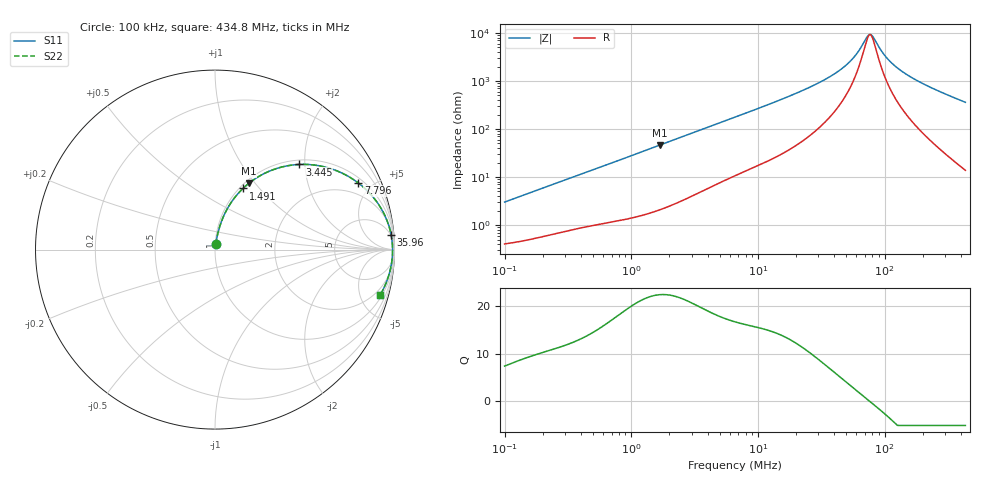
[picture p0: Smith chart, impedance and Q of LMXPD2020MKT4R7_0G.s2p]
! LMXPD2020MKT4R7_0G  S-PARAMETER MODEL  ( General Type )
! Model Generated by TAIYO YUDEN Corporation (http://www.ty-top.com)
! Version 1.0
! TAIYO YUDEN Control No. 191023NI43SB-FBB
! Copyright(c) 2019 TAIYO YUDEN CO.,LTD. All Rights Reserved.
! Product Description (link to TY-COMPAS)
! https://ds.yuden.co.jp/TYCOMPAS/or/detail?pn=LMXPD2020MKT4R7M0G&u=M
! Products Name : Inductors
! Characteristics :
!  Inductance : 4.7 uH , SRF(min) : -Hz , DC Resistance(max) : 0.39 Ohm
!  Rated Current : Saturation :1100 mA , Temp Rise : 750 mA
!  Case Size : 2.0 x 2.0 / 0.079 x 0.079 [mm/inch] , Thickness : 1.2 / 0.047 [mm/inch]
!  (Conditions: Temperature = 25 degC , DC Bias Current/Voltage = 0A / 0V)
! External Node Assignments :
!  1  o---GGG---o  2
! GND o---------o GND
! Frequency Range : 0.1MHz  -  434.768421MHz  [ 402 STEP ]
# MHz S RI R 50
! Freq[MHz].  S11 Real  S11 Imag  S21 Real  S21 Imag  S12 Real  S12 Imag  S22 Real  S22 Imag
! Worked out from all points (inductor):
!   401 points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, 100 kHz to 434.8 MHz, reference 50 ohm
!   read as one part in series: L = 4.73 uH near 104.3 kHz
!   highest Q = 22.3 at 1.69 MHz (marker M1), where L = 4.38 uH
!   self-resonance near 76.44 MHz
!   S11 on the Smith chart (normalised r, x): 100 kHz: 1.01, +0.06; 1.491 MHz: 1.04, +0.82; 3.445 MHz: 1.09, +1.87; 7.796 MHz: 1.26, +4.16; 35.96 MHz: 4, +23; 434.8 MHz: 1.28, -7.19
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0.1  0.00491 0.0296  0.9951 -0.0296  0.9951 -0.0296  0.00491 0.0296
0.406826  0.0216 0.1123  0.9784 -0.1123  0.9784 -0.1123  0.0216 0.1123
0.864672  0.0653 0.2218  0.9347 -0.2218  0.9347 -0.2218  0.0653 0.2218
1.490521  0.1557 0.3406  0.8443 -0.3406  0.8443 -0.3406  0.1557 0.3406
1.65507  0.1829 0.3648  0.8171 -0.3648  0.8171 -0.3648  0.1829 0.3648
1.690099  0.1888 0.3696  0.8112 -0.3696  0.8112 -0.3696  0.1888 0.3696
3.4448  0.4694 0.4744  0.5306 -0.4744  0.5306 -0.4744  0.4694 0.4744
6.733248  0.7518 0.4028  0.2482 -0.4028  0.2482 -0.4028  0.7518 0.4028
7.796401  0.7981 0.3715  0.2019 -0.3715  0.2019 -0.3715  0.7981 0.3715
13.43943  0.9138 0.2482  0.0862 -0.2482  0.0862 -0.2482  0.9138 0.2482
26.82484  0.972 0.1217  0.028 -0.1217  0.028 -0.1217  0.972 0.1217
35.96468  0.9815 0.0817  0.0185 -0.0817  0.0185 -0.0817  0.9815 0.0817
53.54187  0.9877 0.0365  0.0123 -0.0365  0.0123 -0.0365  0.9877 0.0365
61.99591  0.9887 0.0214  0.0113 -0.0214  0.0113 -0.0214  0.9887 0.0214
71.78481  0.9893 0.0067  0.0107 -0.0067  0.0107 -0.0067  0.9893 0.0067
76.43979  0.9894 0.000467  0.0106 -0.000467  0.0106 -0.000467  0.9894 0.000467
81.39662  0.9894 -0.00577  0.0106 0.00577  0.0106 0.00577  0.9894 -0.00577
96.24353  0.989 -0.0226  0.011 0.0226  0.011 0.0226  0.989 -0.0226
109.1303  0.9883 -0.0355  0.0117 0.0355  0.0117 0.0355  0.9883 -0.0355
134.5556  0.9861 -0.0584  0.0139 0.0584  0.0139 0.0584  0.9861 -0.0584
180.4018  0.9805 -0.0945  0.0195 0.0945  0.0195 0.0945  0.9805 -0.0945
434.7684  0.9199 -0.2529  0.0801 0.2529  0.0801 0.2529  0.9199 -0.2529
